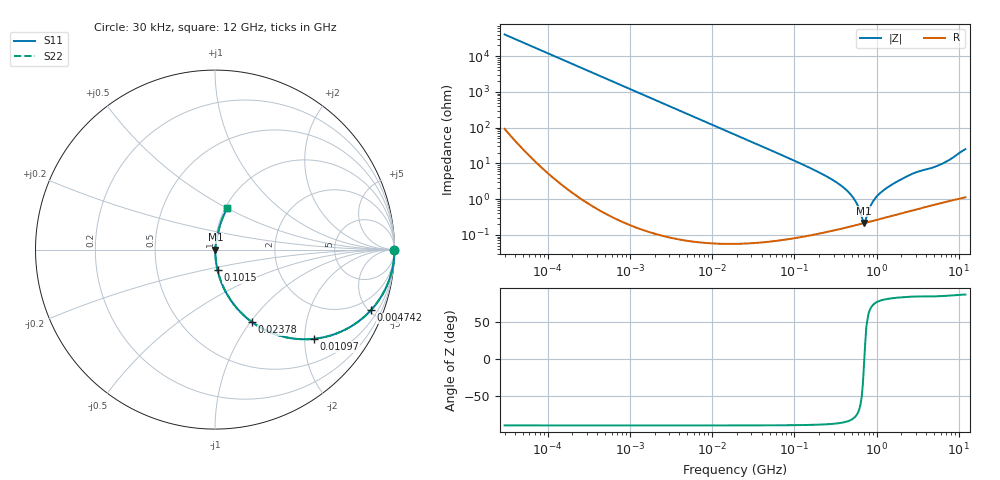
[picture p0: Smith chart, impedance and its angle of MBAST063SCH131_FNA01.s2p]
! MBAST063SCH131_FNA01  S-PARAMETER MODEL  ( General Type )
! Model Generated by TAIYO YUDEN Corporation (http://www.ty-top.com)
! Version 1.0
! TAIYO YUDEN Control No. 130801
! Copyright(c) 2013 TAIYO YUDEN CO.,LTD. All Rights Reserved.
! Product Description (link to TY-COMPAS)
! https://ds.yuden.co.jp/TYCOMPAS/or/detail?pn=MBAST063SCH131JFNA01&u=M
! Products Name : Multilayer Ceramic Capacitors
! Characteristics :
!  Capacitance : 130 pF , Rated Voltage : 25V , TCC : CH / C0H
!  Case Size : 0.6 x 0.3 / 0.024 x 0.012 [mm/inch] , Thickness : 0.3 / 0.012 [mm/inch]
!  (Conditions: Temperature = 25 degC , DC Bias Current/Voltage = 0A / 0V)
! External Node Assignments :
!  1  o---| |---o  2
! GND o---------o GND
! Frequency Range : 0.03MHz  -  12000MHz  [ 401 STEP ]
# MHz S RI R 50
! Freq[MHz].  S11 Real  S11 Imag  S21 Real  S21 Imag  S12 Real  S12 Imag  S22 Real  S22 Imag
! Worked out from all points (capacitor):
!   401 points, 30 kHz to 12 GHz, reference 50 ohm
!   read as one part in series: C = 131 pF near 32 kHz
!   lowest |Z| = 215 mohm at 702.6 MHz (marker M1)
!   series resonance near 707.8 MHz, so ESL is about 390 pH
!   S11 on the Smith chart (normalised r, x): 30 kHz: open; 4.742 MHz: 1.00, -5.14; 10.97 MHz: 1.00, -2.22; 23.78 MHz: 1.00, -1.02; 101.5 MHz: 1.00, -0.24; 12 GHz: 1.02, +0.50
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0.03  1 -0.00246  1.17e-05 0.00246  1.17e-05 0.00246  1 -0.00246
0.260295  0.9995 -0.0214  0.000461 0.0214  0.000461 0.0214  0.9995 -0.0214
2.258455  0.9668 -0.1792  0.0332 0.1792  0.0332 0.1792  0.9668 -0.1792
4.741653  0.8684 -0.3379  0.1316 0.3379  0.1316 0.3379  0.8684 -0.3379
10.96639  0.5524 -0.497  0.4476 0.497  0.4476 0.497  0.5524 -0.497
18.97367  0.2919 -0.4542  0.7081 0.4542  0.7081 0.4542  0.2919 -0.4542
23.77866  0.2079 -0.4052  0.7921 0.4052  0.7921 0.4052  0.2079 -0.4052
43.88187  0.0716 -0.2567  0.9284 0.2567  0.9284 0.2567  0.0716 -0.2567
101.489  0.0144 -0.1158  0.9856 0.1158  0.9856 0.1158  0.0144 -0.1158
164.6252  0.00586 -0.0696  0.9941 0.0696  0.9941 0.0696  0.00586 -0.0696
303.8045  0.0024 -0.0326  0.9976 0.0326  0.9976 0.0326  0.0024 -0.0326
447.3588  0.00191 -0.0163  0.9981 0.0163  0.9981 0.0163  0.00191 -0.0163
560.6502  0.00194 -0.00811  0.9981 0.00811  0.9981 0.00811  0.00194 -0.00811
658.7456  0.00206 -0.00252  0.9979 0.00252  0.9979 0.00252  0.00206 -0.00252
702.6322  0.00213 -0.000225  0.9979 0.000225  0.9979 0.000225  0.00213 -0.000225
749.4426  0.00222 0.0021  0.9978 -0.0021  0.9978 -0.0021  0.00222 0.0021
852.6267  0.00243 0.00636  0.9976 -0.00636  0.9976 -0.00636  0.00243 0.00636
939.2353  0.00262 0.00939  0.9974 -0.00939  0.9974 -0.00939  0.00262 0.00939
1428.372  0.00377 0.0228  0.9962 -0.0228  0.9962 -0.0228  0.00377 0.0228
2722.352  0.00741 0.0508  0.9926 -0.0508  0.9926 -0.0508  0.00741 0.0508
6296.196  0.0173 0.096  0.9827 -0.096  0.9827 -0.096  0.0173 0.096
12000  0.0687 0.2314  0.9313 -0.2314  0.9313 -0.2314  0.0687 0.2314
